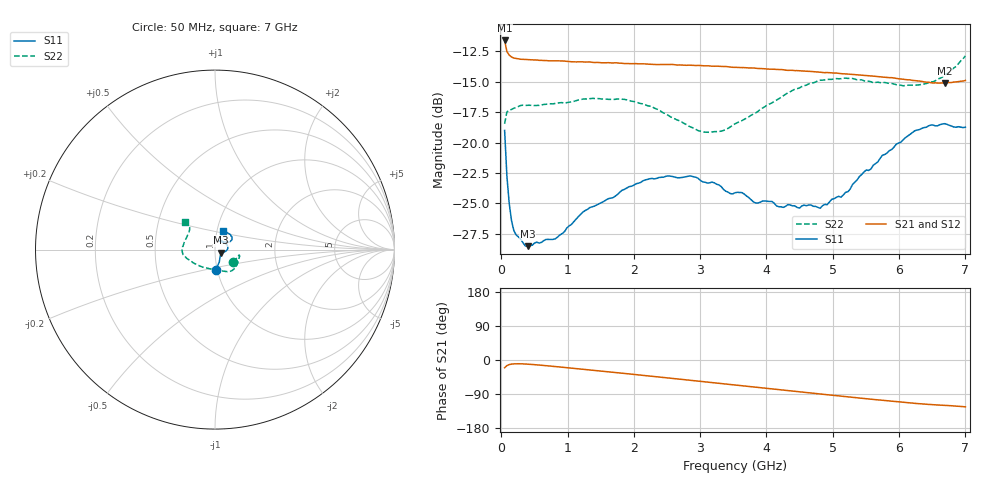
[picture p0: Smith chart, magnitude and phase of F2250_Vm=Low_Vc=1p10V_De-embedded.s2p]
! Integrated Device Technology
! Corporate Headquarters
! 6024 Silver Creek Valley Road
! San Jose, CA 95138  USA
! Phone:  1-408-284-8200
! Toll Free:  1-800-223-1366
! Webpage:  http://www.idt.com/
! Timing and RF Division
! 515 Groton Road, Suite 102
! Westford, MA 01886-6024
! Device:  F2250
! Description: Voltage Variable RF Attenuator
! Frequency:  50.0 -  6000.00 MHz
! Package:  3x3 mm Thin QFN Plastic Package: 16 pin
! Ports:  2 RF, 3 DC
!  Pin  1  = GND
!  Pin  2  = NC
!  Pin  3  = RF1  = Port 1
!  Pin  4  = NC
!  Pin  5  = GND
!  Pin  6  = GND
!  Pin  7  = GND
!  Pin  8  = GND
!  Pin  9  = NC
!  Pin 10  = RF2  = Port 2
!  Pin 11  = NC
!  Pin 12  = GND
!  Pin 13  = GND
!  Pin 14  = VCNTRL
!  Pin 15  = VDD
!  Pin 16  = VMODE
! Vcntrl:  1.100 Volts
! Vmode:  +0.000 Volts
! Vdd:  +3.30  Volts
! Current:  1.192 mA
! Data:  The device was measured on a the F2250 evaluation board which has
!  individual transmission lines to the RF pins.  Data was collected
!  using a calibrated network analyzer.  The evaluation board was
!  de-embedded using a TRL calibration technique.
!  The reference plane is the edge of the package pin.
! Misc:  SN 10
!  Action Tracker AT0258
! Date Measured:  2014-11-26
! Date:  2015-10-15  MJV
! Note:
!  Integrated Device Technology supplies this data as a sample of measured
!  data at the package pin for this product.  Your particular data for this
!  product may vary.
!  Data was taken at 25 degrees C.
!  Integrated Device Technology reserves the right to change this data at anytime.
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# GHz S dB R 50
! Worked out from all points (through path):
!   201 points, 50 MHz to 7 GHz, reference 50 ohm
!   highest |S21| = -11.60 dB at 50 MHz (marker M1); lowest = -15.1 dB at 6.687 GHz (marker M2)
!   group delay of S21, straight-line fit = 48.9 ps
!   lowest |S11| = -28.5 dB at 397.5 MHz (marker M3), VSWR 1.08, Z = 53.4 - j1.76 ohm
!   |S11| at or under -10 dB: start of sweep to end of sweep
!   |S22| runs from -19.2 to -12.9 dB; largest |S21 - S12| = 0.00073
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0.05  -19.00 -87.0  -11.60 -20.5  -11.60 -20.5  -18.46 -34.7
0.08475  -22.79 -70.7  -12.51 -14.8  -12.50 -14.8  -17.48 -19.0
0.1195  -25.02 -61.4  -12.80 -12.1  -12.81 -12.2  -17.34 -14.4
0.15425  -26.44 -54.1  -12.96 -10.8  -12.96 -10.8  -17.28 -13.1
0.22375  -27.61 -40.4  -13.08 -9.9  -13.08 -9.9  -17.11 -13.2
0.3975  -28.54 -26.0  -13.17 -10.9  -13.18 -10.9  -16.93 -15.2
0.8145  -27.94 -17.3  -13.27 -17.3  -13.28 -17.3  -16.78 -27.7
1.2315  -25.73 -15.5  -13.36 -24.4  -13.37 -24.4  -16.42 -38.8
1.857  -23.86 -4.6  -13.50 -35.5  -13.48 -35.5  -16.45 -51.7
2.37825  -22.88 7.0  -13.58 -44.8  -13.56 -44.9  -17.31 -63.9
2.86475  -22.76 21.3  -13.63 -53.8  -13.63 -53.8  -18.74 -84.0
3.0385  -23.24 27.3  -13.69 -57.0  -13.68 -57.0  -19.12 -94.1
3.3165  -23.62 37.7  -13.73 -62.2  -13.72 -62.2  -19.07 -112.4
3.525  -24.14 43.8  -13.81 -66.0  -13.81 -66.0  -18.46 -125.1
3.83775  -24.99 55.4  -13.89 -71.8  -13.88 -71.8  -17.56 -141.3
4.7065  -25.26 59.7  -14.16 -87.8  -14.17 -87.8  -15.08 -169.7
4.81075  -25.41 55.5  -14.21 -89.7  -14.23 -89.7  -14.87 -171.4
5.1235  -24.50 45.5  -14.33 -95.4  -14.35 -95.4  -14.74 -178.5
5.85325  -20.67 28.4  -14.66 -108.2  -14.65 -108.3  -15.14 164.0
6.2355  -19.04 31.1  -14.90 -114.3  -14.90 -114.4  -15.29 151.3
6.68725  -18.45 45.7  -15.11 -119.7  -15.09 -119.7  -14.42 138.5
7  -18.74 66.4  -14.89 -123.6  -14.88 -123.7  -12.87 138.1
